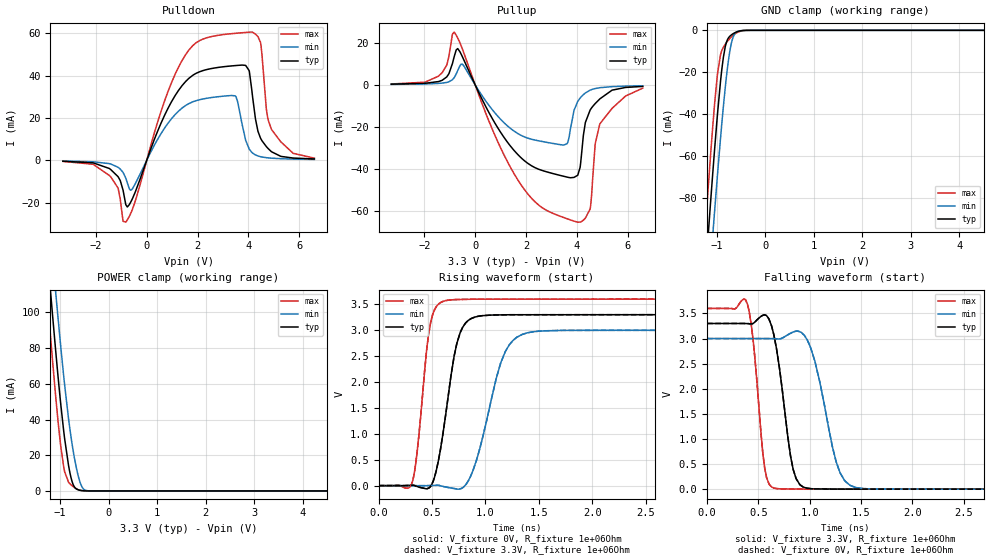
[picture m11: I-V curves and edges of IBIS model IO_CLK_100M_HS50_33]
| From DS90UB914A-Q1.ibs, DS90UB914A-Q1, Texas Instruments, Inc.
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|   Model IO_CLK_100M_HS50_33
[Model]   IO_CLK_100M_HS50_33
Model_type   I/O
Polarity   Non-Inverting
Enable   Active-Low
Vinl = 0.8
Vinh = 2
Vmeas = 1.65
Vref = 3.3
Cref = 1pF
Rref = 1000000
|   typ   min   max
C_comp   1.107pF   1.107pF   1.107pF
[Voltage Range]   3.3   3   3.6
[Temperature Range]   25   105   -40
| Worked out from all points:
|   slope of the pulldown table from 0 to 0.495 V, typ, clamps not added: 31.7 ohm
|   slope of the pullup table from 0 to 0.495 V, typ, clamps not added: 40.7 ohm
|   GND clamp passes 1 mA (typ) near -0.61 V on its own axis
|   POWER clamp passes 1 mA (typ) near -0.66 V on its own axis
|   falling waveform, V_fixture 3.3V, R_fixture 1e+06Ohm: 20-80 % time 125ps typ, 183ps min, 90ps max; typ from 3.3 V to 0 V
|   rising waveform, V_fixture 0V, R_fixture 1e+06Ohm: 20-80 % time 146ps typ, 218ps min, 101ps max; typ from 0 V to 3.3 V
|   rising waveform, V_fixture 3.3V, R_fixture 1e+06Ohm: 20-80 % time 146ps typ, 218ps min, 101ps max; typ from 0 V to 3.3 V
|   falling waveform, V_fixture 0V, R_fixture 1e+06Ohm: 20-80 % time 125ps typ, 183ps min, 90ps max; typ from 3.3 V to 0 V
[Pulldown]
|   Voltage   I(typ)   I(min)   I(max)
-3.3V     -492uA     -370.1uA   -562.4uA
-1.429V   -4.316mA   -1.75mA    -7.71mA
-825mV    -20.99mA   -8.467mA   -29.28mA
-587.4mV  -18.75mA   -13.84mA   -23.88mA
699.6mV   21.18mA    15.14mA    27.98mA
1.521V    37.08mA    25.79mA    49.74mA
3.472V    44.68mA    30.41mA    59.92mA
4.036V    41.74mA    5.147mA    60.5mA
4.471V    10.47mA    1.66mA     55.73mA
4.709V    6.339mA    1.184mA    23.64mA
4.907V    3.978mA    956.3uA    14.5mA
6.59V     584uA      365.9uA    967.5uA
[GND Clamp]
|   Voltage   I(typ)   I(min)   I(max)
-3.3V     -824.9mA   -829.6mA   -826.6mA
-1.231V   -115mA     -143.7mA   -92.78mA
-1.122V   -80.3mA    -109.8mA   -57.66mA
-1.082V   -68.1mA    -97.7mA    -45.69mA
-1.053V   -59.17mA   -88.76mA   -37.21mA
-983.4mV  -39.45mA   -68.41mA   -20.45mA
-924mV    -24.55mA   -51.81mA   -11.74mA
-864.6mV  -12.91mA   -36.42mA   -8.1mA
-805.2mV  -5.979mA   -22.89mA   -6.014mA
-716.1mV  -2.493mA   -8.014mA   -3.527mA
-567.6mV  -570.3uA   -496.4uA   -912.8uA
6.59V     0A         0A         0A
[Pullup]
|   Voltage   I(typ)   I(min)   I(max)
-3.3V     328.6uA    226.5uA    421.1uA
-1.449V   1.569mA    698.9uA    4.127mA
-825mV    13.48mA    3.456mA    25.19mA
-498.3mV  13.29mA    9.825mA    16.96mA
1.759V    -34.24mA   -23.78mA   -46.86mA
3.61V     -43.98mA   -28.12mA   -63.84mA
4.036V    -43.02mA   -7.85mA    -65.5mA
4.333V    -17.94mA   -3.846mA   -63.57mA
4.521V    -11.99mA   -2.507mA   -59.2mA
4.719V    -8.918mA   -1.747mA   -28.13mA
4.907V    -6.634mA   -1.34mA    -18.53mA
6.59V     -734uA     -424.5uA   -1.559mA
[POWER Clamp]
|   Voltage   I(typ)   I(min)   I(max)
-3.3V     833.5mA    841.2mA    832.9mA
-1.33V    155.7mA    186.6mA    131.8mA
-1.251V   129.7mA    161.4mA    105mA
-1.221V   120.1mA    152.1mA    95.13mA
-1.152V   98.01mA    130.6mA    72.56mA
-1.092V   79.64mA    112.5mA    54.11mA
-924mV    33.68mA    64.51mA    13.53mA
-775.5mV  7.783mA    30.77mA    3.49mA
-636.9mV  740.9uA    9.827mA    892.9uA
-547.8mV  166.8uA    2.302mA    194.3uA
-409.2mV  6.208uA    51.74uA    5.076uA
6.59V     0A         0A         0A
[Ramp]
R_load = 1e+06
|   typ   min   max
dV/dt_r   1.97992/1.45968e-10   1.79991/2.17902e-10   2.15993/1.00998e-10
dV/dt_f   1.97994/1.25048e-10   1.79993/1.83361e-10   2.15995/8.99813e-11
[Falling Waveform]
V_fixture = 3.3V
V_fixture_min = 3V
V_fixture_max = 3.6V
R_fixture = 1e+06Ohm
C_fixture = 0F
|   Time   V(typ)   V(min)   V(max)
0s        3.3V       3V         3.6V
392.6ps   3.298V     3V         3.69V
448.4ps   3.302V     3V         2.972V
561.3ps   3.472V     3V         417.1mV
652.1ps   3.056V     2.998V     22.01mV
813.8ps   649.2mV    3.106V     3.515mV
937.1ps   41.45mV    3.084V     1.817mV
1.258ns   1.603mV    540.3mV    797.3uV
1.443ns   829.3uV    35.55mV    760uV
4.8ns     97.08uV    115.1uV    82.84uV
[Rising Waveform]
V_fixture = 0V
V_fixture_min = 0V
V_fixture_max = 0V
R_fixture = 1e+06Ohm
C_fixture = 0F
|   Time   V(typ)   V(min)   V(max)
0s        5.185uV    -3.245uV   1.228uV
312.8ps   7.265mV    2.552uV    56.14mV
466.9ps   -47.72mV   1.42mV     2.916V
605.3ps   1.052V     -15.9mV    3.557V
705.7ps   2.492V     -55.24mV   3.588V
786.2ps   3.055V     -39.92mV   3.593V
916.8ps   3.261V     497.6mV    3.598V
1.143ns   3.295V     2.369V     3.598V
1.343ns   3.298V     2.917V     3.599V
4.8ns     3.3V       3V         3.6V
[Rising Waveform]
V_fixture = 3.3V
V_fixture_min = 3V
V_fixture_max = 3.6V
R_fixture = 1e+06Ohm
C_fixture = 0F
|   Time   V(typ)   V(min)   V(max)
0s        100uV      115.5uV    80.28uV
312.8ps   7.36mV     121.2uV    56.28mV
466.9ps   -47.56mV   1.538mV    2.916V
605.3ps   1.053V     -15.78mV   3.557V
705.7ps   2.492V     -55.05mV   3.589V
786.2ps   3.055V     -39.63mV   3.593V
916.8ps   3.261V     498.2mV    3.598V
1.143ns   3.295V     2.37V      3.599V
1.343ns   3.298V     2.917V     3.599V
4.8ns     3.3V       3V         3.6V
[Falling Waveform]
|Gnd
V_fixture = 0V
V_fixture_min = 0V
V_fixture_max = 0V
R_fixture = 1e+06Ohm
C_fixture = 0F
|   Time   V(typ)   V(min)   V(max)
0s        3.3V       3V         3.6V
392.6ps   3.297V     3V         3.69V
448.4ps   3.302V     3V         2.971V
561.3ps   3.471V     3V         416.8mV
652.1ps   3.055V     2.998V     21.91mV
813.8ps   648.7mV    3.106V     3.433mV
937.1ps   41.31mV    3.084V     1.737mV
1.258ns   1.506mV    539.7mV    717.8uV
1.443ns   733.2uV    35.38mV    680.5uV
4.8ns     2.223uV    -3.665uV   3.712uV
